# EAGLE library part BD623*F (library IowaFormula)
H-bridge driver for brush motors Source: http://www.rohm.com/products/databook/motor/pdf/bd623x_series-e.pdf
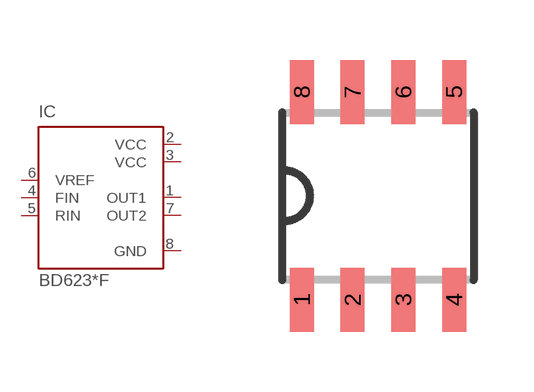
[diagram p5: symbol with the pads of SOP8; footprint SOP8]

Designator prefix IC

## BD6230F (MPN: BD6230F-E2; OC_FARNELL: 1716264; OC_NEWARK: 15R0529), BD6231F (MPN: BD6231F-E2; OC_FARNELL: 1716265; OC_NEWARK: 15R0530)  [SOP8]
1  OUT1  out
2  VCC  pwr
3  VCC  pwr
4  FIN  in
5  RIN  in
6  VREF  pas
7  OUT2  out
8  GND  pwr

## Footprint SOP8 (pad centres in mm)
SOP8 Source: http://www.rohm.com/products/databook/motor/pdf/bd623x_series-e.pdf
smd 0.6 x 1.6: 1 -1.905,-2.6; 2 -0.635,-2.6; 3 0.635,-2.6; 4 1.905,-2.6; 5 1.905,2.6; 6 0.635,2.6; 7 -0.635,2.6; 8 -1.905,2.6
